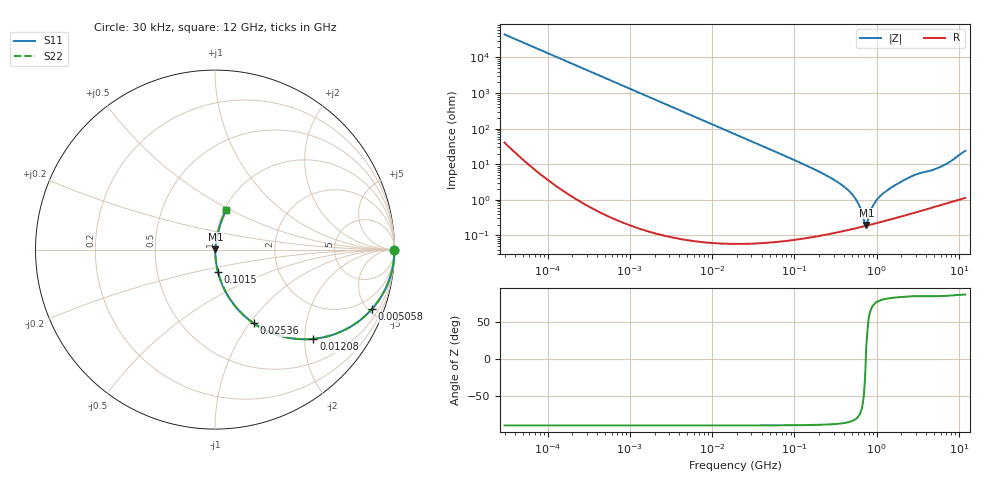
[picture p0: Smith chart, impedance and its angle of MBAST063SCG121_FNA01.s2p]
! MBAST063SCG121_FNA01  S-PARAMETER MODEL  ( General Type )
! Model Generated by TAIYO YUDEN Corporation (http://www.ty-top.com)
! Version 1.0
! TAIYO YUDEN Control No. 130801
! Copyright(c) 2013 TAIYO YUDEN CO.,LTD. All Rights Reserved.
! Product Description (link to TY-COMPAS)
! https://ds.yuden.co.jp/TYCOMPAS/or/detail?pn=MBAST063SCG121JFNA01&u=M
! Products Name : Multilayer Ceramic Capacitors
! Characteristics :
!  Capacitance : 120 pF , Rated Voltage : 25V , TCC : CG / C0G
!  Case Size : 0.6 x 0.3 / 0.024 x 0.012 [mm/inch] , Thickness : 0.3 / 0.012 [mm/inch]
!  (Conditions: Temperature = 25 degC , DC Bias Current/Voltage = 0A / 0V)
! External Node Assignments :
!  1  o---| |---o  2
! GND o---------o GND
! Frequency Range : 0.03MHz  -  12000MHz  [ 401 STEP ]
# MHz S RI R 50
! Freq[MHz].  S11 Real  S11 Imag  S21 Real  S21 Imag  S12 Real  S12 Imag  S22 Real  S22 Imag
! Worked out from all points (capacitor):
!   401 points, 30 kHz to 12 GHz, reference 50 ohm
!   read as one part in series: C = 120 pF near 32 kHz
!   lowest |Z| = 196 mohm at 749.4 MHz (marker M1)
!   series resonance near 738.8 MHz, so ESL is about 390 pH
!   S11 on the Smith chart (normalised r, x): 30 kHz: open; 5.058 MHz: 1.00, -5.26; 12.08 MHz: 1.00, -2.20; 25.36 MHz: 1.00, -1.05; 101.5 MHz: 1.00, -0.26; 12 GHz: 1.02, +0.48
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0.03  1 -0.00225  7.14e-06 0.00225  7.14e-06 0.00225  1 -0.00225
0.260295  0.9996 -0.0195  0.000385 0.0195  0.000385 0.0195  0.9996 -0.0195
2.258455  0.972 -0.1649  0.028 0.1649  0.028 0.1649  0.972 -0.1649
5.057549  0.8738 -0.332  0.1262 0.332  0.1262 0.332  0.8738 -0.332
12.08034  0.5482 -0.4974  0.4518 0.4974  0.4518 0.4974  0.5482 -0.4974
18.97367  0.3296 -0.4697  0.6704 0.4697  0.6704 0.4697  0.3296 -0.4697
25.36282  0.2158 -0.4108  0.7842 0.4108  0.7842 0.4108  0.2158 -0.4108
45.32004  0.0793 -0.2692  0.9207 0.2692  0.9207 0.2692  0.0793 -0.2692
101.489  0.017 -0.1264  0.983 0.1264  0.983 0.1264  0.017 -0.1264
164.6252  0.00674 -0.0763  0.9933 0.0763  0.9933 0.0763  0.00674 -0.0763
313.7612  0.00238 -0.0347  0.9976 0.0347  0.9976 0.0347  0.00238 -0.0347
462.0203  0.00174 -0.0175  0.9983 0.0175  0.9983 0.0175  0.00174 -0.0175
579.0248  0.00169 -0.0089  0.9983 0.0089  0.9983 0.0089  0.00169 -0.0089
637.8412  0.00173 -0.00536  0.9983 0.00536  0.9983 0.00536  0.00173 -0.00536
702.6322  0.0018 -0.00188  0.9982 0.00188  0.9982 0.00188  0.0018 -0.00188
749.4426  0.00186 0.000609  0.9981 -0.000609  0.9981 -0.000609  0.00186 0.000609
880.5704  0.00208 0.00572  0.9979 -0.00572  0.9979 -0.00572  0.00208 0.00572
970.0175  0.00224 0.00865  0.9978 -0.00865  0.9978 -0.00865  0.00224 0.00865
1428.372  0.00314 0.0201  0.9969 -0.0201  0.9969 -0.0201  0.00314 0.0201
2722.352  0.00631 0.0464  0.9937 -0.0464  0.9937 -0.0464  0.00631 0.0464
6502.545  0.0157 0.0902  0.9843 -0.0902  0.9843 -0.0902  0.0157 0.0902
12000  0.0632 0.2206  0.9368 -0.2206  0.9368 -0.2206  0.0632 0.2206
